PROGRAM MAIN
VAR
	Master                 :axis_Ref;
	Slave                  :axis_Ref;
	
	state                  : FlyingState;
	
	(*Power Part*)
	PowerMaster            : MC_Power;
	PowerMasterOut         : ST_McOutputs;
	PowerSlave             : MC_Power;
	PowerSlaveOut          : ST_McOutputs;
	PowerEnable            : BOOL;
	
	(*Reset Part*)
	ResetMaster			   : MC_Reset;
	ResetMasterOut		   : ST_McOutputs;
	ResetSlave			   : MC_Reset;
	ResetSlaveOut		   : ST_McOutputs;
	
	(*Move Axes Part*)
	MoveMaster			   : MC_MoveVelocity;
	MoveMasterOut		   : ST_McOutputs;
	MoveSlave			   : MC_MoveAbsolute;
	MoveSlaveOut		   : ST_McOutputs;
	HaltSlave			   : MC_Halt;
	HaltSlaveOut		   : ST_McOutputs;
	
	(*FlyingSaw Part*)
	GearInPos			   : MC_GearInPos;
	GearInPosOut		   : ST_McOutputs;
	GearOut				   : MC_GearOut;
	GearOutOut			   : ST_McOutputs;	
	StartSync              : BOOL;
	
	(*Timing Part*)
	Ton_SyncTime           : TON;
END_VAR

VAR CONSTANT
	Master_V               : LREAL:=433;
	SlaveMax_V             : LREAL:=533;
	MasterSync_P           : LREAL:= 500;
	SlaveSync_P            : LREAL:= 500;
	PREFERCONSTANTVELOCITY : BOOL:=TRUE;
	ENABLECHECKS           : BOOL:=FALSE;
	SyncTime               : TIME:=T#5S;
	
END_VAR

(*update all axes status*)
Master();
Slave();
CASE state OF 
	F_INIT:
	(*reset all funtion blocks*)
		ResetMaster.Execute := FALSE;
		ResetSlave.Execute := FALSE;
		MoveMaster.Execute := FALSE;
		MoveSlave.Execute := FALSE;
		GearInPos.Execute := FALSE;
		GearOut.Execute := FALSE;
		state:=F_ENABLE;
	F_ENABLE:
		PowerEnable:=TRUE;
		IF PowerMaster.Status AND PowerSlave.Status THEN
			state:=F_PREPARE1;
		ELSIF PowerMaster.Error OR PowerSlave.Error THEN
			state:=F_ERROR;
		END_IF
	F_PREPARE1:
	(*Start Master Axis*)
		MoveMaster.Velocity:=Master_V;
		MoveMaster.Execute:=TRUE;
		IF MoveMaster.InVelocity THEN
			State:=F_PREPARE2;
		ELSIF MoveMaster.CommandAborted OR MoveMaster.Error THEN
			State:=F_ERROR;
		END_IF
	F_PREPARE2:
	(*calculate synchronization parameters*)
		GearOut.Execute:=FALSE;
		GearInPos.Execute:=FALSE;
		GearInPos.Velocity:=SlaveMax_V;
		GearInPos.MasterSyncPosition:=MasterSync_P;
		GearInPos.SlaveSyncPosition :=SlaveSync_P;
		(* activate checks *)
		GearInPos.SyncMode.GearInSync_OpMask_IgnoreMasterAcc := TRUE;	                (* master acceleration is not useful if the master is an encoder axis *)
		GearInPos.SyncMode.GearInSync_OpMask_PreferConstVelo := PREFERCONSTANTVELOCITY; (* the synchronization will try to accelerate fast and get into constant velocity phase *)
		IF ENABLECHECKS THEN
			GearInPos.SyncMode.GearInSync_CheckMask_MaxPos := TRUE; 	                 (* check position limits *)
			GearInPos.SyncMode.GearInSync_CheckMask_MinPos := TRUE; 	                 (* check position limits *)
			GearInPos.SyncMode.GearInSync_CheckMask_MaxVelo := TRUE; 	                 (* check velocity limits *)
			GearInPos.SyncMode.GearInSync_CheckMask_MaxAcc := FALSE; 	                 (* don't check acceleration limits *)
			GearInPos.SyncMode.GearInSync_CheckMask_MaxDec := FALSE;	                 (* don't check acceleration limits *)
;		END_IF
		state:=F_COUPLE;
	F_COUPLE:
	(*wait for master and slave to be synchronized*)
		GearInPos.Execute:=TRUE;
		IF GearInPos.InSync THEN
			state:=F_SYNCHRONIZED;
		ELSIF GearInPos.CommandAborted OR GearInPos.Error THEN
			state:=F_ERROR;
		END_IF
	F_SYNCHRONIZED:
	(*master and slave in synchronized motion*)
		Ton_SyncTime.IN:=TRUE;
		Ton_SyncTime.PT:=SyncTime;
		IF Ton_SyncTime.Q THEN
			state:=F_DECOUPLE;
		END_IF
	F_DECOUPLE:
	(*gear out-slave will keep its velocity *)
	GearOut.Execute:= TRUE;
			IF  GearOut.Error THEN
				GearOut.Execute:= TRUE;
				state := F_ERROR;
			END_IF	
	F_ERROR:
		GearOut.Execute:= Slave.Status.Coupled; (* gear out if done already *)
		IF Master.Status.Error OR Slave.Status.Error  THEN
			state := F_RESET;	(* axis error requires reset *)
		ELSE
			state := F_INIT;		(* function block errors don't need a reset *)
		END_IF

	F_RESET :
		ResetMaster.Execute := TRUE;
		ResetSlave.Execute := TRUE;
		IF ResetMaster.Done AND ResetSlave.Done  THEN
			state := F_INIT;
		ELSIF ResetMaster.Error OR ResetSlave.Error  THEN
			state := F_INIT; (* can't do anything here *)
		END_IF	
END_CASE

ACTPOWER();
ACTFLYINGSAW();
ACTMOVE();
ACTRESET();

ACTION ACTFLYINGSAW:
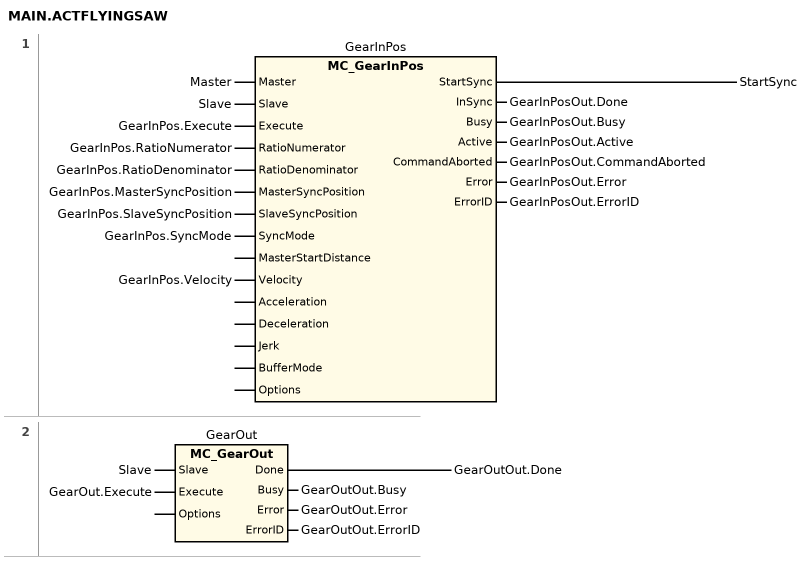
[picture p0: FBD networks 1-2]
// NETWORK 1
GearInPos(
    Master := Master,
    Slave := Slave,
    Execute := GearInPos.Execute,
    RatioNumerator := GearInPos.RatioNumerator,
    RatioDenominator := GearInPos.RatioDenominator,
    MasterSyncPosition := GearInPos.MasterSyncPosition,
    SlaveSyncPosition := GearInPos.SlaveSyncPosition,
    SyncMode := GearInPos.SyncMode,
    Velocity := GearInPos.Velocity,
    InSync => GearInPosOut.Done,
    Busy => GearInPosOut.Busy,
    Active => GearInPosOut.Active,
    CommandAborted => GearInPosOut.CommandAborted,
    Error => GearInPosOut.Error,
    ErrorID => GearInPosOut.ErrorID); // MC_GearInPos
StartSync := GearInPos.StartSync;

// NETWORK 2
GearOut(
    Slave := Slave,
    Execute := GearOut.Execute,
    Busy => GearOutOut.Busy,
    Error => GearOutOut.Error,
    ErrorID => GearOutOut.ErrorID); // MC_GearOut
GearOutOut.Done := GearOut.Done;
END_ACTION

ACTION ACTMOVE:
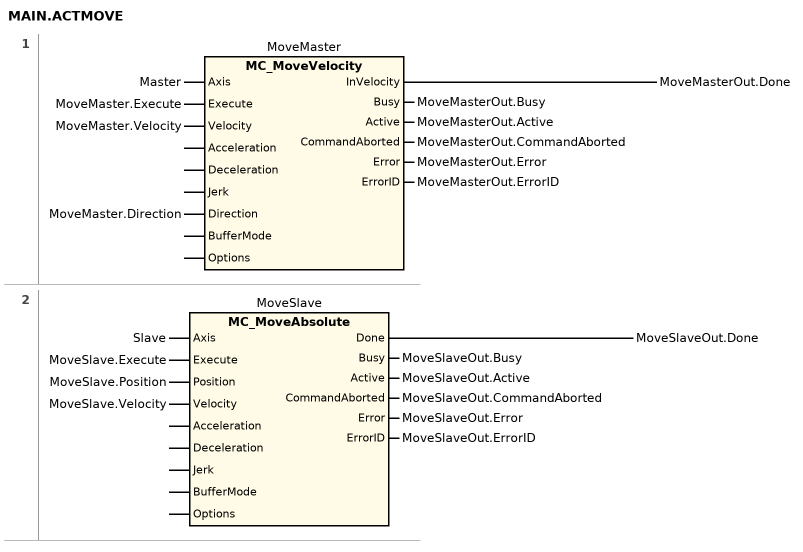
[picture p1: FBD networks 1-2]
// NETWORK 1
MoveMaster(
    Axis := Master,
    Execute := MoveMaster.Execute,
    Velocity := MoveMaster.Velocity,
    Direction := MoveMaster.Direction,
    Busy => MoveMasterOut.Busy,
    Active => MoveMasterOut.Active,
    CommandAborted => MoveMasterOut.CommandAborted,
    Error => MoveMasterOut.Error,
    ErrorID => MoveMasterOut.ErrorID); // MC_MoveVelocity
MoveMasterOut.Done := MoveMaster.InVelocity;

// NETWORK 2
MoveSlave(
    Axis := Slave,
    Execute := MoveSlave.Execute,
    Position := MoveSlave.Position,
    Velocity := MoveSlave.Velocity,
    Busy => MoveSlaveOut.Busy,
    Active => MoveSlaveOut.Active,
    CommandAborted => MoveSlaveOut.CommandAborted,
    Error => MoveSlaveOut.Error,
    ErrorID => MoveSlaveOut.ErrorID); // MC_MoveAbsolute
MoveSlaveOut.Done := MoveSlave.Done;
END_ACTION

ACTION ACTPOWER:
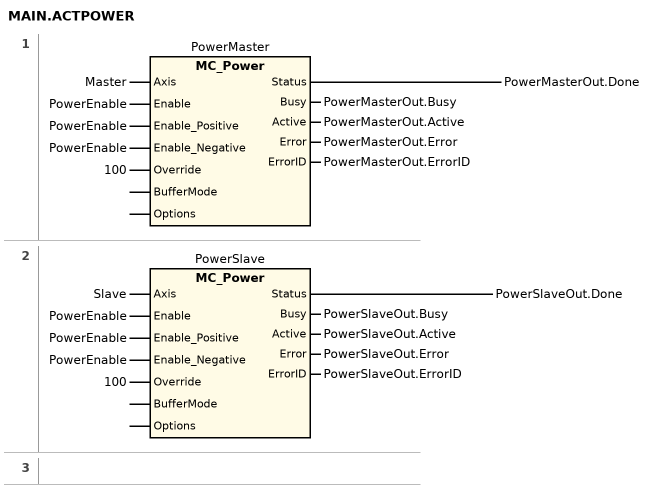
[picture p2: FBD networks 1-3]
// NETWORK 1
PowerMaster(
    Axis := Master,
    Enable := PowerEnable,
    Enable_Positive := PowerEnable,
    Enable_Negative := PowerEnable,
    Override := 100,
    Busy => PowerMasterOut.Busy,
    Active => PowerMasterOut.Active,
    Error => PowerMasterOut.Error,
    ErrorID => PowerMasterOut.ErrorID); // MC_Power
PowerMasterOut.Done := PowerMaster.Status;

// NETWORK 2
PowerSlave(
    Axis := Slave,
    Enable := PowerEnable,
    Enable_Positive := PowerEnable,
    Enable_Negative := PowerEnable,
    Override := 100,
    Busy => PowerSlaveOut.Busy,
    Active => PowerSlaveOut.Active,
    Error => PowerSlaveOut.Error,
    ErrorID => PowerSlaveOut.ErrorID); // MC_Power
PowerSlaveOut.Done := PowerSlave.Status;

// NETWORK 3
END_ACTION

ACTION ACTRESET:
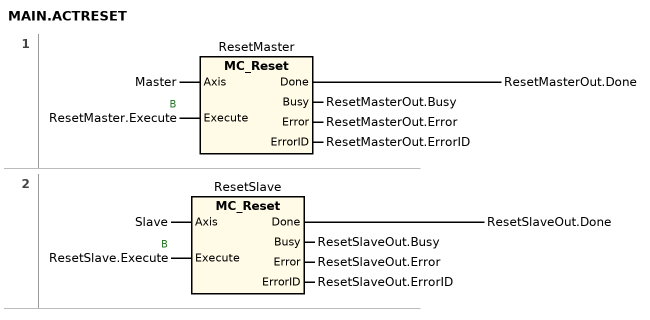
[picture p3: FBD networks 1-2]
// NETWORK 1
//   ResetMaster.Execute: B
ResetMaster(
    Axis := Master,
    Execute := ResetMaster.Execute,
    Busy => ResetMasterOut.Busy,
    Error => ResetMasterOut.Error,
    ErrorID => ResetMasterOut.ErrorID); // MC_Reset
ResetMasterOut.Done := ResetMaster.Done;

// NETWORK 2
//   ResetSlave.Execute: B
ResetSlave(
    Axis := Slave,
    Execute := ResetSlave.Execute,
    Busy => ResetSlaveOut.Busy,
    Error => ResetSlaveOut.Error,
    ErrorID => ResetSlaveOut.ErrorID); // MC_Reset
ResetSlaveOut.Done := ResetSlave.Done;
END_ACTION

END_PROGRAM
